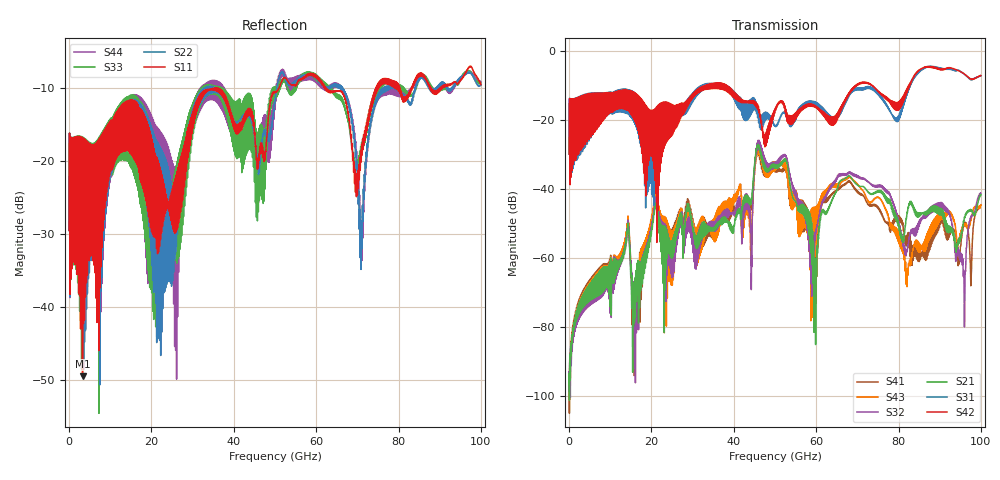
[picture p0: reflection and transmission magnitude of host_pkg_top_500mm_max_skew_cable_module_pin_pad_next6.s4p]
# Hz S RI R 50
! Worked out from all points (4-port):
!   10000 points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, 10 MHz to 100 GHz, reference 50 ohm
!   strongest paths, dB at 10 MHz, 25.01 GHz, 50.01 GHz, 75.01 GHz, 100 GHz:
!     S42: -29.9, -15.8, -16.8, -11.6, -7.2
!     S31: -29.9, -18.2, -21.7, -12.7, -7.2
!     S21: -96.7, -58.5, -33.2, -40.7, -41.8
!     S32: -96.3, -59.5, -32.9, -39.4, -41.5
!     S43: -96.7, -55.4, -32.6, -42.5, -44.7
!     S41: -97.2, -55.9, -33.4, -45.2, -44.6
!   lowest |S11| = -49.5 dB at 3.27 GHz (marker M1), VSWR 1.01, Z = 50.2 + j0.295 ohm
!   |S11| at or under -10 dB: start of sweep to 35.62 GHz; 35.62 GHz to 50.97 GHz (15.35 GHz wide, 35.5 % of centre); 62.26 GHz to 74.55 GHz (12.29 GHz wide, 18 % of centre)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
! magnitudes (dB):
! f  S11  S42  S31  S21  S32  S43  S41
! 10 MHz  -29.5  -29.9  -29.9  -96.7  -96.3  -96.7  -97.2
! 3.27 GHz  -49.5  -24.8  -22.5  -72.4  -73.2  -71.9  -71.2
! 46.09 GHz  -19.2  -17.9  -18.9  -27.4  -26.1  -28.1  -29.7
! 59.69 GHz  -8.4  -16.2  -15.7  -71.4  -52.7  -47.5  -58.6
! 67.71 GHz  -13.5  -12.6  -13.4  -36.3  -35.7  -36.9  -37.8
! 95.87 GHz  -8.3  -6.6  -6.7  -49.4  -65.0  -50.0  -50.8
! 100 GHz  -9.5  -7.2  -7.2  -41.8  -41.5  -44.7  -44.6
